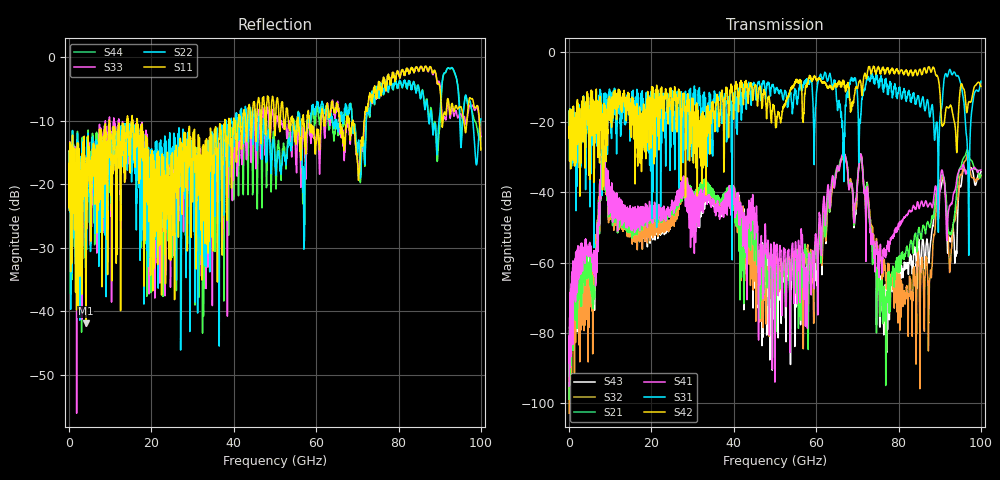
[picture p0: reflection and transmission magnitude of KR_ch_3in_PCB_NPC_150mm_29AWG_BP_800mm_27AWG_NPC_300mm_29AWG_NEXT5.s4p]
# GHz S RI R 45
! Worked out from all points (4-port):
!   4000 points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, 25 MHz to 100 GHz, reference 45 ohm
!   strongest paths, dB at 25 MHz, 25.02 GHz, 50.02 GHz, 75.03 GHz, 100 GHz:
!     S42: -21.3, -17.5, -18.0, -4.3, -9.8
!     S31: -21.3, -12.1, -11.4, -8.0, -8.3
!     S41: -95.3, -43.6, -84.8, -61.6, -33.6
!     S21: -99.0, -44.8, -64.1, -61.7, -35.0
!     S32: -103.0, -47.1, -68.8, -60.0, -35.3
!     S43: -97.7, -47.3, -67.9, -61.4, -34.1
!   lowest |S11| = -41.8 dB at 4.075 GHz (marker M1), VSWR 1.02, Z = 44.6 - j0.582 ohm
!   |S11| at or under -10 dB: start of sweep to 9.799 GHz; 9.805 GHz to 14.12 GHz (4.314 GHz wide, 36.1 % of centre); 16.58 GHz to 37.83 GHz (21.26 GHz wide, 78.1 % of centre)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
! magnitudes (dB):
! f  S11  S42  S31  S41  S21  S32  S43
! 25 MHz  -16.7  -21.3  -21.3  -95.3  -99.0  -103.0  -97.7
! 4.075 GHz  -41.8  -23.1  -34.9  -55.3  -61.9  -67.1  -60.3
! 8.25 GHz  -17.0  -18.7  -17.5  -28.1  -28.8  -28.8  -28.1
! 48.33 GHz  -6.5  -12.9  -8.5  -55.0  -63.2  -65.0  -69.6
! 70.78 GHz  -15.5  -8.4  -19.1  -29.2  -29.9  -29.7  -29.0
! 76.6 GHz  -3.4  -5.9  -9.8  -58.2  -70.9  -61.2  -69.0
! 100 GHz  -14.6  -9.8  -8.3  -33.6  -35.0  -35.3  -34.1
